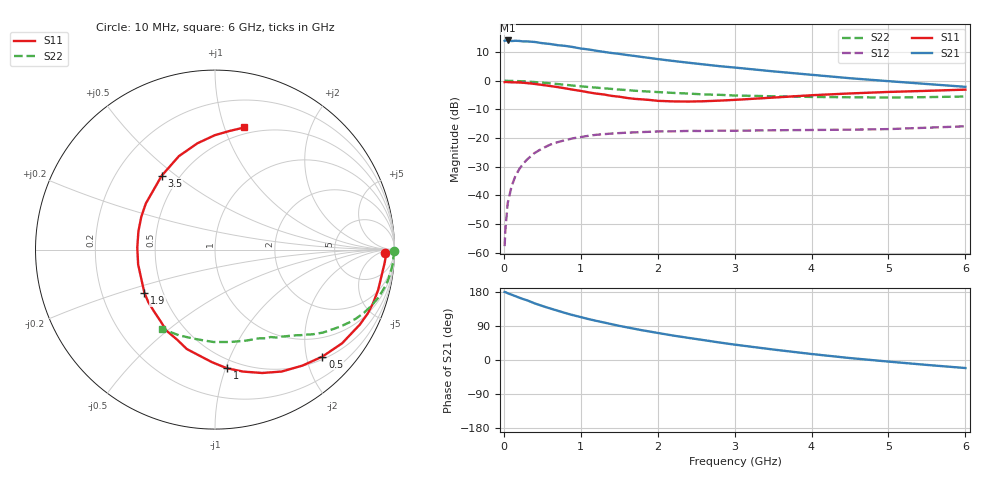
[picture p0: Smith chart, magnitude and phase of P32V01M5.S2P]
! SIEMENS Small Signal Semiconductors
! BFP181
! Si NPN RF Bipolar Junction Transistor in SOT143
! VCE = 2 V  IC = 1.5 mA
! Common Emitter S-Parameters:  March  1996
# GHz  S  MA  R  50
!  f  S11  S21  S12  S22
! GHz  MAG  ANG  MAG  ANG  MAG  ANG  MAG  ANG
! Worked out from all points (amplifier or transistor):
!   36 points, 10 MHz to 6 GHz, reference 50 ohm
!   highest |S21| = 14.1 dB at 50 MHz (marker M1)
!   |S21| within 3 dB of that: start of sweep to 1.058 GHz
!   unconditionally stable (mu >= 1): 2.646 GHz to end of sweep
!   at 250 MHz: K = 0.11, MSG = 21.4 dB, |S12| = -29.0 dB
!   at 1.4 GHz: K = 0.58, MSG = 14.0 dB, |S12| = -18.4 dB
!   at 6 GHz: K = 1.21, MAG = 4.1 dB, |S12| = -15.9 dB
!   S11 on the Smith chart (normalised r, x): 10 MHz: 32, -11; 500 MHz: 0.55, -2.31; 1 GHz: 0.43, -1.01; 1.9 GHz: 0.39, -0.24; 3.5 GHz: 0.40, +0.45; 6 GHz: 0.44, +1.17
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0.01  0.9452 -1.1  4.975 179.5  0.0013 96.7  0.9985 -0.4
0.02  0.953 -1.8  5.026 179.1  0.0025 82.9  0.9999 -0.9
0.05  0.9482 -4.4  5.043 176.2  0.0073 88.0  0.9951 -2.2
0.1  0.939 -9.2  4.928 172.4  0.0143 83.4  0.9945 -4.2
0.15  0.9364 -13.9  4.98 168.5  0.0218 80.4  0.9889 -6.3
0.2  0.9301 -18.7  4.944 164.6  0.0287 78.9  0.9828 -8.5
0.3  0.9086 -27.4  4.854 157.7  0.0421 72.9  0.9688 -12.4
0.4  0.8796 -36.4  4.747 149.5  0.0549 67.7  0.9493 -16.3
0.5  0.8446 -44.9  4.524 142.6  0.0659 62.1  0.9256 -19.8
0.6  0.8093 -53.0  4.379 136.2  0.0765 57.7  0.9016 -23.0
0.8  0.7359 -69.1  4.05 123.9  0.0922 49.1  0.8497 -28.6
0.9  0.6975 -77.0  3.868 118.3  0.099 45.3  0.8226 -31.2
1  0.6647 -84.2  3.648 113.2  0.1041 42.1  0.7989 -33.4
1.1  0.6277 -91.5  3.514 108.0  0.1095 39.0  0.7777 -35.5
1.5  0.5266 -120.9  2.943 90.1  0.1221 29.1  0.7012 -42.4
1.9  0.4612 -148.5  2.49 75.0  0.1288 22.3  0.6453 -48.1
2.2  0.4361 -169.1  2.215 64.5  0.131 18.6  0.6133 -52.2
2.8  0.4497 156.0  1.798 46.3  0.1344 13.3  0.568 -60.5
3.5  0.5079 125.7  1.458 27.7  0.1368 9.8  0.5358 -71.3
4.5  0.6003 99.4  1.106 5.1  0.1401 6.6  0.5149 -91.0
5.5  0.6664 82.9  0.877 -13.0  0.1516 7.2  0.5179 -112.5
6  0.6997 76.5  0.783 -21.2  0.1605 6.1  0.5305 -123.5
